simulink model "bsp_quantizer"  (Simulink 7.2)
settings: Solver=ode45  StartTime=0.0  StopTime=10.0  RelTol=1e-3
StopFcn:
  | bsp_quantizer_plot

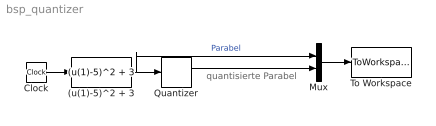
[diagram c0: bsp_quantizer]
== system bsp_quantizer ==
  note: quantisierte Parabel
  (u(1)-5)^2 + 3 : Fcn  Expr=(u(1)-5)^2 + 3
  Clock : Clock
  Mux : Mux  Inputs=2
  Quantizer : Quantizer  QuantizationInterval=5
  To Workspace : ToWorkspace  VariableName=ausgabe  SampleTime=-1  SaveFormat=Array
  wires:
  Clock/1 -> (u(1)-5)^2 + 3/1
  Quantizer/1 -> Mux/2
  Mux/1 -> To Workspace/1
  (u(1)-5)^2 + 3/1 -> Quantizer/1, Mux/1  "Parabel"
